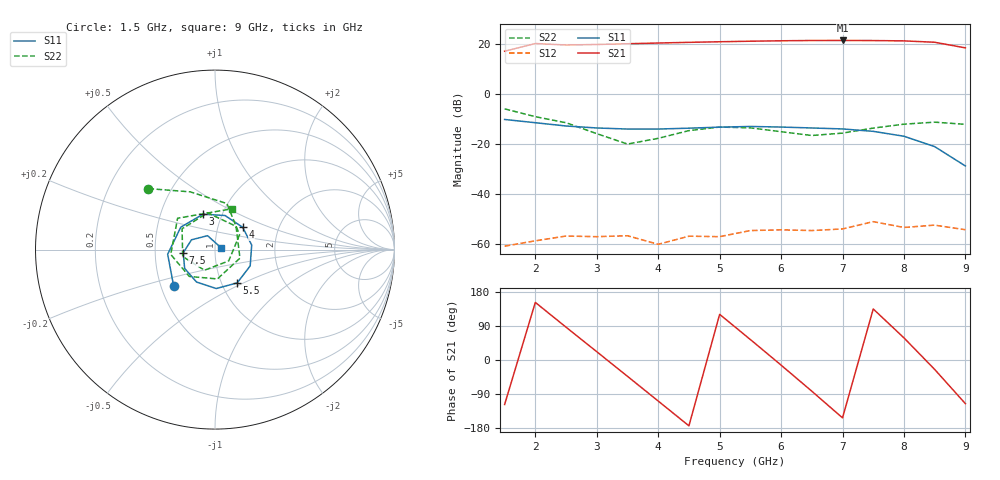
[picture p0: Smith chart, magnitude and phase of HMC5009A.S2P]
! HMMC-5009 S Parameters
! (VD1=VD2=4.5V, VD3=VD4=7.0V, ID1+ID2=180mA (VG1=VG2), ID3+ID4=400 mA (VG3=VG4),
# ghz s ma r 50
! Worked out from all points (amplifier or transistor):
!   16 points, 1.5 GHz to 9 GHz, reference 50 ohm
!   highest |S21| = 21.4 dB at 7 GHz (marker M1)
!   |S21| within 3 dB of that: 1.713 GHz to end of sweep
!   unconditionally stable (mu >= 1): start of sweep to end of sweep
!   at 2.5 GHz: K = 32.52, MAG = 20.2 dB, |S12| = -57.0 dB
!   at 5.5 GHz: K = 21.79, MAG = 21.6 dB, |S12| = -54.8 dB
!   at 9 GHz: K = 29.48, MAG = 18.7 dB, |S12| = -54.4 dB
!   S11 on the Smith chart (normalised r, x): 1.5 GHz: 0.58, -0.26; 3 GHz: 0.81, +0.33; 4 GHz: 1.31, +0.34; 5.5 GHz: 1.18, -0.46; 7.5 GHz: 0.70, -0.03; 9 GHz: 1.07, +0.02
1.5  0.308 -138.3  7.18 -117.4  0.00089 76.1  0.503 137.5
2  0.265 -174.4  10.24 152.0  0.00114 36.7  0.35 113.2
2.5  0.228 146.7  9.56 86.6  0.00142 -1.3  0.265 75.5
3  0.208 108.7  9.8 21.9  0.00138 -17.7  0.16 31.2
3.5  0.198 73.6  10.14 -43.1  0.00144 -46.0  0.099 -39.6
4  0.198 38.9  10.48 -108.3  0.00097 -56.8  0.129 -117.0
4.5  0.206 7.1  10.82 -173.7  0.00141 -72.7  0.184 -167.9
5  0.216 -24.8  11.11 120.5  0.00138 -105.1  0.217 147.7
5.5  0.223 -56.3  11.4 54.0  0.00183 -102.8  0.209 101.4
6  0.217 -88.1  11.62 -13.5  0.00189 -142.8  0.175 48.0
6.5  0.208 -119.6  11.78 -82.3  0.00183 -174.2  0.147 -18.9
7  0.199 -148.2  11.8 -152.7  0.00197 146.3  0.164 -85.3
7.5  0.178 -174.2  11.74 134.7  0.00276 121.0  0.207 -133.7
8  0.142 157.4  11.57 58.4  0.00211 97.9  0.248 -173.7
8.5  0.088 118.2  10.86 -24.9  0.00235 57.7  0.272 140.0
9  0.036 15.6  8.38 -115.2  0.0019 26.4  0.246 67.5
